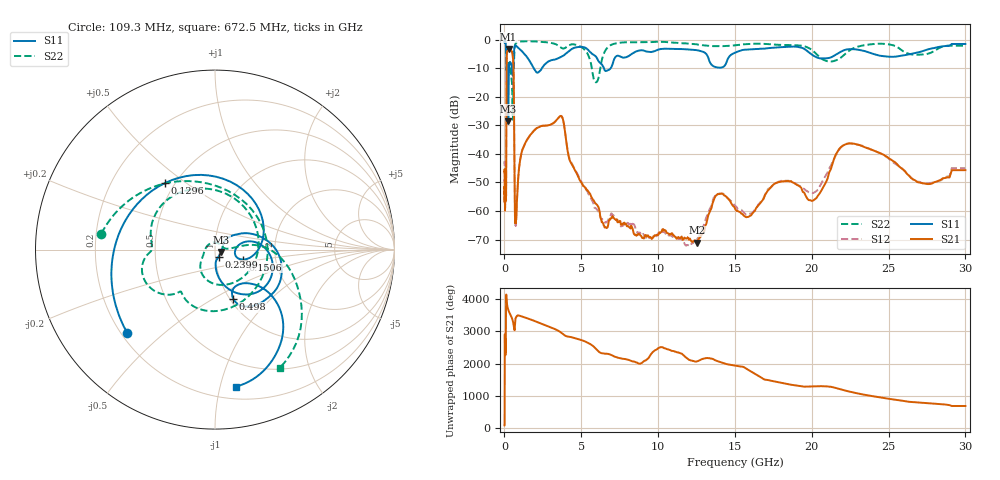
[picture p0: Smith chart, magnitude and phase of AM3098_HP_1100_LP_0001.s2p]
! Date/Time: Thu, Feb 28, 2019 8:44 AM
! Network Analyzer: Agilent Technologies E8364B Rev: A.07.50.67
! Sweep from 0.010 to 30.000 GHz, 1601 Points, Sweep Type: LOG
! Power Supply: 5.023 V, 0.002 A
# Hz S DB R 50
!freq MagS11 AngS11 MagS21 AngS21 MagS12 AngS12 MagS22 AngS22
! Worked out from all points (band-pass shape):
!   1601 points, 10 MHz to 30 GHz, reference 50 ohm
!   highest |S21| = -3.31 dB at 265.1 MHz (marker M1); lowest = -71.1 dB at 12.56 GHz (marker M2)
!   |S21| within 3 dB of the highest: 148.6 MHz to 551.1 MHz (402.5 MHz wide, 115 % of centre)
!   lowest |S11| = -28.6 dB at 246 MHz (marker M3), VSWR 1.08, Z = 53.6 - j1.48 ohm
!   |S11| at or under -10 dB: 204.5 MHz to 301.1 MHz (96.59 MHz wide, 38.2 % of centre); 1.898 GHz to 2.441 GHz (543.2 MHz wide, 25 % of centre); 6.472 GHz to 6.92 GHz (448 MHz wide, 6.69 % of centre)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
!   |S22| runs from -28.1 to -0.5 dB; largest |S21 - S12| = 0.012
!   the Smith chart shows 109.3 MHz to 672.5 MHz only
!   S11 on the Smith chart (normalised r, x): 109.3 MHz: 0.22, -0.38; 129.6 MHz: 0.44, +0.42; 150.6 MHz: 1.36, -0.16; 239.9 MHz: 1.04, -0.08; 498 MHz: 1.04, -0.62; 672.5 MHz: 0.29, -1.12
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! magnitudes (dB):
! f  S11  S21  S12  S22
! 10 MHz  -0.4  -46.4  -43.7  -0.5
! 38.04 MHz  -0.4  -57.1  -56.4  -0.7
! 109.3 MHz  -3.4  -52.1  -54.0  -3.9
! 129.6 MHz  -6.7  -21.4  -21.4  -10.5
! 144.7 MHz  -11.8  -7.5  -7.5  -9.4
! 150.6 MHz  -15.6  -5.9  -5.8  -10.2
! 201.3 MHz  -9.6  -3.9  -3.8  -7.5
! 239.9 MHz  -27.0  -3.4  -3.3  -9.0
! 246 MHz  -28.6  -3.3  -3.3  -9.1
! 265.1 MHz  -17.3  -3.3  -3.3  -9.0
! 498 MHz  -10.7  -4.4  -4.4  -16.6
! 550.5 MHz  -12.1  -6.3  -6.2  -27.8
! 605.4 MHz  -5.6  -15.6  -15.6  -11.6
! 672.5 MHz  -2.2  -58.1  -56.1  -2.5
! 735.8 MHz  -2.1  -64.2  -65.2  -1.3
! 2.084 GHz  -11.5  -31.1  -31.1  -0.7
! 3.704 GHz  -6.0  -26.8  -26.8  -2.9
! 5.959 GHz  -6.0  -57.5  -59.2  -15.0
! 7.926 GHz  -6.2  -64.6  -63.7  -1.0
! 12.56 GHz  -3.8  -71.1  -69.6  -1.7
! 22.56 GHz  -3.4  -36.4  -36.3  -3.5
! 30 GHz  -1.6  -45.7  -45.0  -2.1
